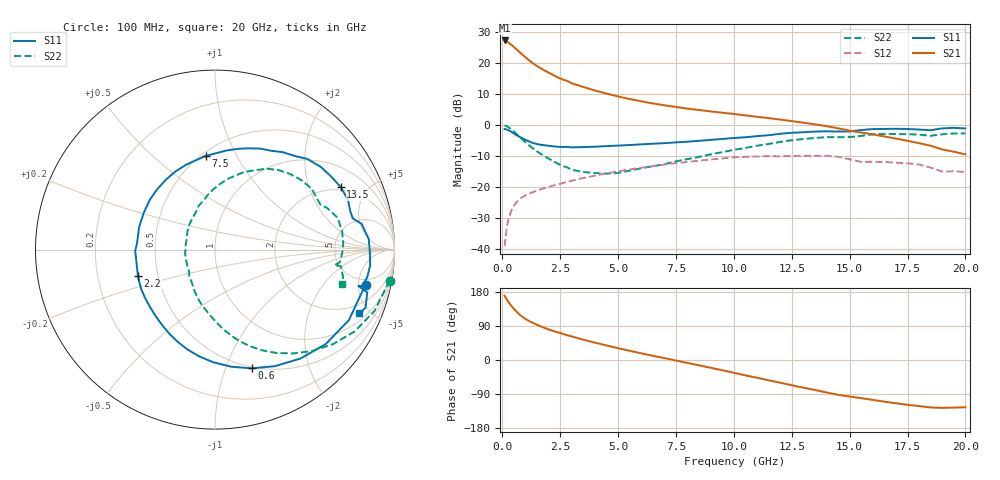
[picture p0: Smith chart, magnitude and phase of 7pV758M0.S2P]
! Infineon Technologies  Discrete & RF Semiconductors
! bfp620
! VCE = 0.75 V,  IC =  8.0 mA
! Common Emitter S-Parameters:  Sep 2002
# GHz  S  MA  R  50
!  f  S11  S21  S12  S22
! GHz  MAG  ANG  MAG  ANG  MAG  ANG  MAG  ANG
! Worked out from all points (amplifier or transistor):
!   59 points, 100 MHz to 20 GHz, reference 50 ohm
!   highest |S21| = 27.2 dB at 100 MHz (marker M1)
!   |S21| within 3 dB of that: start of sweep to 634.2 MHz
!   unconditionally stable (mu >= 1): 4.34 GHz to 10.76 GHz; 16.91 GHz to end of sweep
!   at 1 GHz: K = 0.44, MSG = 22.2 dB, |S12| = -22.7 dB
!   at 5.5 GHz: K = 1.05, MAG = 10.0 dB, |S12| = -14.3 dB
!   at 20 GHz: K = 1.53, MAG = -1.4 dB, |S12| = -15.1 dB
!   S11 on the Smith chart (normalised r, x): 100 MHz: 4.03, -6.09; 600 MHz: 0.49, -1.23; 2.2 GHz: 0.38, -0.14; 7.5 GHz: 0.53, +0.76; 13.5 GHz: 1.83, +3.30; 20 GHz: 1.38, -4.33
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0.1  0.861 -13.1  22.92 169.6  0.0112 83.1  0.9877 -10.1
0.2  0.8432 -27.8  21.96 159.3  0.0236 75.8  0.9523 -21.0
0.3  0.8108 -40.5  20.73 150.3  0.0339 69.6  0.902 -30.3
0.4  0.7709 -52.0  19.37 142.3  0.0425 64.3  0.8435 -38.6
0.5  0.7302 -62.8  17.99 135.0  0.0499 59.7  0.7828 -46.2
0.6  0.6923 -72.9  16.66 128.4  0.0562 55.8  0.7236 -53.1
0.7  0.6584 -82.2  15.42 122.5  0.0616 52.5  0.6681 -59.5
0.9  0.6014 -98.5  13.23 112.5  0.0701 47.5  0.5707 -70.3
1  0.5769 -105.5  12.29 108.4  0.0736 45.6  0.5286 -74.9
1.2  0.5353 -117.8  10.67 101.5  0.0796 42.7  0.4565 -82.8
1.4  0.5043 -128.4  9.4 95.7  0.085 40.7  0.399 -89.7
1.7  0.4775 -142.3  8.001 87.8  0.0929 38.5  0.3352 -99.6
2.2  0.4538 -161.2  6.363 76.6  0.1058 35.6  0.2618 -115.2
3  0.4357 175.2  4.682 62.4  0.1265 31.0  0.1899 -139.4
3.5  0.4409 163.6  4.097 53.5  0.1401 27.8  0.175 -154.3
5  0.4656 133.7  2.879 31.2  0.1796 16.9  0.1689 158.5
7  0.5093 102.1  2.072 5.1  0.2304 0.2  0.2333 117.3
7.5  0.5244 95.6  1.95 -1.5  0.2436 -4.6  0.2598 110.5
10.5  0.6343 60.2  1.427 -40.6  0.307 -36.4  0.4271 74.7
13.5  0.7822 26.5  1.022 -79.1  0.3184 -69.4  0.6178 38.8
17  0.869 -5.8  0.605 -114.2  0.2472 -99.9  0.7155 3.1
20  0.8798 -23.8  0.337 -124.8  0.1752 -112.5  0.7322 -15.0
